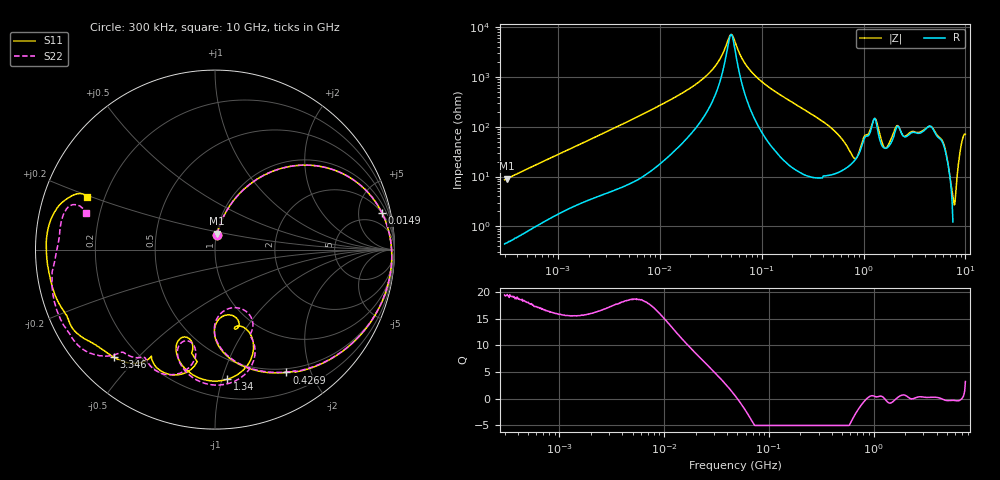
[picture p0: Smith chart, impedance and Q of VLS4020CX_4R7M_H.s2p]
! S-Parameter Data Generated by TDK Corporation
! Copyright(C) 2024 TDK Corporation.
! All Rights Reserved.
! TDK P/N: VLS4020CX-4R7M-H (SMD / SMT Inductor (Coil))
! Property: L=4.7uH at 1MHz
! Size(LxWxT): 4x4x2mm
! Model Type: s2p (Touchstone File Format Version 1.0)
! Frequency: DC=Yes Start=0.3MHz Stop=10000MHz 802points Log-sweep
! Model Generated on May 28, 2024
! Terms and conditions regarding TDK Simulation Models:
! 1)This simulation model is being provided solely for informational
!  purposes. Please refer to the specifications of the products in
!  terms of detailed characteristics of such products.
! 2)In no event shall TDK Corporation of any of its subsidiaries be
!  liable for any loss or damage arising, directly or indirectly,
!  from any information contained in this simulation model, including,
!  but not limited to loss or damages arising from any inaccuracies,
!  omissions or errors in connection with such information.
! 3)Any and all copyrights on this simulation model are owned by
!  TDK Corporation.  Duplication or redistribution of this simulation
!  model without prior written permission from TDK Corporation
!  is prohibited.
! 4)This simulation model is subject to any modification or change
!  without any prior notice.
! 5)Neither TDK Corporation nor any of its subsidiaries shall make any
!  warranty, express or implied, including but not limited to the
!  correctness, implied warranties of merchantability and fitness for
!  a particular purpose with respect to this simulation models.
! 6)The use of this simulation model shall be deemed to have consented
!  to the terms and conditions hereof.
! Port Assignments:
!  1 ---@@@--- 2
! Applicable Conditions:
!  Temperature = 25 degC
!  DC Bias Current = 0 A
!  Small Signal Operation
# Hz S MA R 50
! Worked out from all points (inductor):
!   801 points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, 300 kHz to 10 GHz, reference 50 ohm
!   read as one part in series: L = 4.53 uH near 318.3 kHz
!   highest Q = 19.4 at 318.3 kHz (marker M1), where L = 4.55 uH
!   self-resonance near 50.17 MHz
!   S11 on the Smith chart (normalised r, x): 300 kHz: 1.01, +0.17; 14.9 MHz: 2.01, +8.87; 426.9 MHz: 0.45, -1.65; 1.34 GHz: 0.34, -1.04; 3.346 GHz: 0.11, -0.43; 10 GHz: 0.13, +0.19
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300000  0.08479 82.0  0.9921 -4.9  0.9918 -4.9  0.08486 82.1
318337  0.08978 81.8  0.9913 -5.2  0.9913 -5.2  0.0899 81.8
1713600  0.4085 62.2  0.887 -24.2  0.887 -24.2  0.4085 62.2
9671944  0.9123 20.1  0.3544 -66.2  0.3544 -66.2  0.9123 20.1
1.49005e7  0.953 12.2  0.2294 -72.6  0.2294 -72.6  0.9531 12.3
3.249697e7  0.9813 1.9  0.07181 -75.1  0.07182 -75.1  0.9814 2.0
4.929468e7  0.986 -3.0  0.01418 -14.3  0.01418 -14.3  0.9861 -2.9
5.477226e7  0.9864 -4.3  0.01941 42.0  0.0194 42.0  0.9864 -4.2
9.444554e7  0.9823 -12.3  0.1092 71.7  0.1092 71.7  0.9822 -12.1
3.126428e8  0.8755 -45.9  0.4388 41.5  0.4388 41.5  0.8758 -45.5
4.269249e8  0.7921 -59.8  0.5472 26.3  0.5472 26.3  0.7925 -59.3
7.235338e8  0.5443 -87.4  0.7101 -11.1  0.7101 -11.2  0.5432 -87.1
9.560117e8  0.3784 -75.5  0.6528 -46.1  0.653 -46.1  0.3431 -70.5
1.196827e9  0.5284 -67.2  0.4202 -65.4  0.42 -65.5  0.6042 -68.3
1.339606e9  0.7257 -84.5  0.3068 -43.0  0.3068 -43.0  0.753 -86.0
1.767019e9  0.5239 -110.7  0.5138 -71.1  0.514 -71.1  0.5404 -108.9
2.172958e9  0.7298 -106.9  0.2648 -91.1  0.265 -91.2  0.7306 -107.8
3.34571e9  0.8236 -133.3  0.1884 -115.4  0.1887 -115.5  0.769 -132.0
4.574322e9  0.8976 -148.4  0.08128 -121.5  0.08125 -121.5  0.9185 -142.4
5.76861e9  0.9085 -157.6  0.07823 -115.9  0.07817 -116.0  0.94 -152.4
7.875699e9  0.9407 176.2  0.07007 -133.4  0.06968 -133.3  0.8773 178.8
1e10  0.7718 157.7  0.04997 -127.8  0.05004 -127.8  0.7461 164.0
